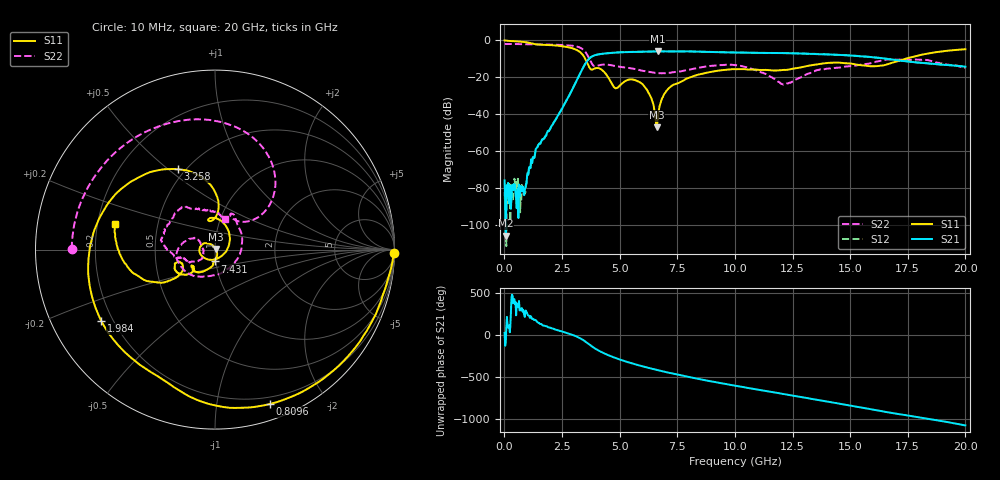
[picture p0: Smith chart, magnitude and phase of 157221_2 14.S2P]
!  2-Port S-parameters saved by WinCal
! VAR MeasName=S-Parameters (CALIBRATED_DATA) read from VNA (N5242A)
! VAR MeasDate=2015-5-26 16:48:03
! VAR NAME=157221_2 14
! VAR FILENAME=157221_2 14.S2P
! VAR DATE=2015-5-26 16:48:03
! VAR PHYS_PORTS=1,2
# Hz S DB R 50
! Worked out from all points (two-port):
!   801 points, 10 MHz to 20 GHz, reference 50 ohm
!   highest |S21| = -5.95 dB at 6.657 GHz (marker M1); lowest = -105.9 dB at 59.98 MHz (marker M2)
!   |S21| within 3 dB of the highest: 3.772 GHz to 15.8 GHz (12.03 GHz wide, 123 % of centre); 15.80238 GHz to 15.82992 GHz (27.55 MHz wide, 0.174 % of centre)
!   lowest |S11| = -47.2 dB at 6.607 GHz (marker M3), VSWR 1.01, Z = 50.3 + j0.335 ohm
!   |S11| at or under -10 dB: 3.508 GHz to 17.4 GHz (13.89 GHz wide, 133 % of centre)
!   |S22| runs from -24.0 to -2.0 dB; largest |S21 - S12| = 0.0084
!   S11 on the Smith chart (normalised r, x): 10 MHz: open; 809.6 MHz: 0.14, -1.41; 1.984 GHz: 0.16, -0.28; 3.258 GHz: 0.46, +0.54; 7.431 GHz: 0.99, -0.13; 20 GHz: 0.27, +0.12
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1e7  -0.04 -1.1  -76.00 25.1  -82.33 -47.4  -1.96 179.8
5.9975e7  -0.12 -6.3  -105.90 -85.7  -85.18 108.4  -1.96 178.5
8.096e8  -0.79 -70.4  -79.36 -59.8  -79.19 -38.7  -2.02 160.4
1.434288e9  -2.23 -114.6  -57.88 154.9  -57.96 156.4  -2.14 144.4
1.984012e9  -2.53 -148.0  -48.18 87.8  -48.03 87.0  -2.28 128.5
3.258375e9  -6.14 114.9  -18.66 -34.3  -18.64 -34.6  -3.80 68.5
3.358325e9  -7.25 104.1  -16.14 -49.4  -16.13 -49.6  -4.45 60.1
4.082962e9  -15.07 91.0  -7.57 176.4  -7.57 176.1  -13.58 66.0
4.882562e9  -25.79 -72.2  -6.57 81.8  -6.54 81.6  -14.08 53.1
5.932038e9  -23.16 149.4  -6.10 -6.6  -6.11 -6.9  -16.37 11.1
6.6067e9  -47.18 49.6  -5.97 -53.3  -5.98 -53.5  -17.72 -35.0
6.656675e9  -42.89 -21.5  -5.95 -56.7  -5.96 -56.9  -17.74 -39.3
6.681662e9  -39.67 -35.4  -5.95 -58.4  -5.95 -58.6  -17.73 -40.6
6.931538e9  -29.15 -70.4  -5.98 -74.5  -5.97 -74.7  -17.84 -54.5
7.431288e9  -23.61 -92.2  -6.02 -104.7  -5.99 -105.0  -17.08 -82.8
8.655675e9  -17.92 -114.8  -6.19 -173.4  -6.18 -173.6  -14.37 -131.6
1.0005e10  -15.60 -133.6  -6.58 119.4  -6.58 119.0  -13.42 -175.6
1.210395e10  -16.05 -139.1  -6.87 20.6  -6.89 20.0  -24.03 -177.6
1.335332e10  -13.42 -139.0  -7.34 -38.5  -7.30 -38.8  -17.29 -150.9
1.470265e10  -12.30 -157.2  -7.95 -102.6  -7.97 -102.9  -14.35 -166.8
1.667666e10  -12.75 -145.4  -10.17 161.9  -10.16 161.9  -10.31 170.0
2e10  -4.82 165.7  -14.26 7.5  -14.32 5.7  -14.94 71.2
